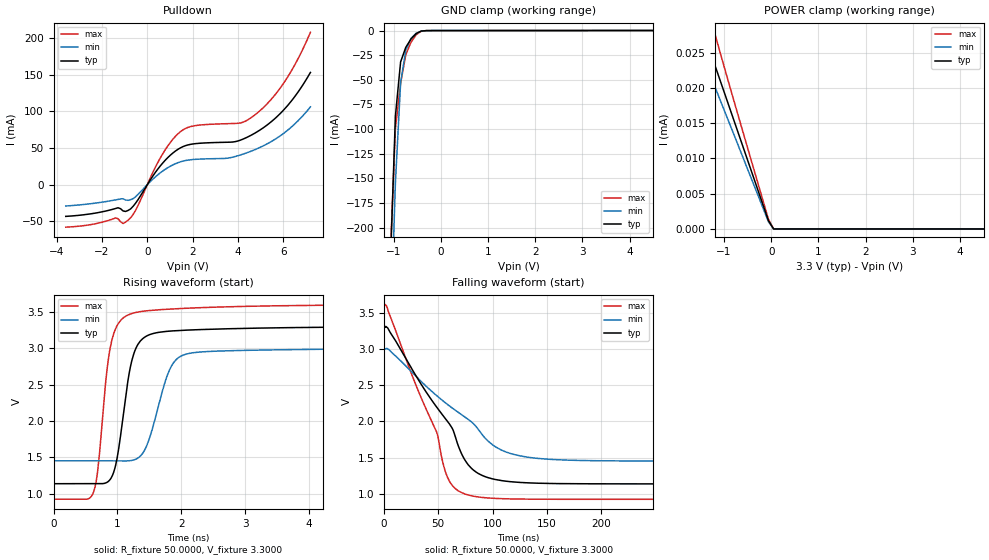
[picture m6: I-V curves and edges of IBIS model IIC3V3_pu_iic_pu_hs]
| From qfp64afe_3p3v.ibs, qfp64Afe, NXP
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[Model] IIC3V3_pu_iic_pu_hs
|   Model IIC3V3_pu_iic_pu_hs
| This model was characterised for following simulation conditions:
| External (pad) voltage:
|   - Typ: 3.3V,   - Min: 3.0V,   - Max: 3.6V
| Library cells for typ/min/max conditions are connected as defined below:
|  IO - External Pad
|  A - Core Input
|  EN - Output Buffer Enable
|  BOOST - vdde
|  ECS - vdd
|  EGP - gnd
|  ENZI - vdd
|  EPD - gnd
|  EPUN - gnd
|  SSEL - vdd
|  ZI - NC
|  ZIF - NC
|  gnd - gnd
|  gnde - gnde
|  vdd - vdd
|  vdde - vdde
| All other pins connected to ground
Model_type I/O_open_drain
Polarity   Non-Inverting
Enable   Active-Low
Vinl =   0.9900V
Vinh =   2.3100V
Vmeas =  1.6500V
Cref =   0.0F
Rref =   1.0000k
Vref =   3.3000V
C_comp   3.5867pF   3.4362pF   3.7352pF
|C_comp_pullup   0.9044pF   0.8908pF   0.9076pF
|C_comp_pulldown   2.3321pF   2.4859pF   2.1859pF
[Model Spec]
| variable   typ   min   max
Vinh   0.9900V   0.9000V   1.0800V
Vinl   2.3100V   2.1000V   2.5200V
Vmeas   1.6500V   1.5000V   1.8000V
Vref   3.3000V   3.0000V   3.6000V
Cref   0.0F   0.0F   0.0F
Rref   1.0000k   1.0000k   1.0000k
[Temperature Range]   25.0000   0.1250k   -40.0000
[Voltage Range]   3.3000V   3.0000V   3.6000V
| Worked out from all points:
|   slope of the pulldown table from 0 to 0.495 V, typ, clamps not added: 22 ohm
|   GND clamp passes 1 mA (typ) near -0.43 V on its own axis
|   rising waveform, R_fixture 50.0000, V_fixture 3.3000: 20-80 % time 227ps typ, 308ps min, 192ps max; typ from 1.14 V to 3.3 V
|   falling waveform, R_fixture 50.0000, V_fixture 3.3000: 20-80 % time 50.8ns typ, 68.7ns min, 38.5ns max; typ from 3.3 V to 1.14 V
[Pulldown]
|Voltage   I(typ)   I(min)   I(max)
-3.6V     -43.22mA   -29.09mA   -57.9mA
-1.29V    -31.46mA   -20.15mA   -46.47mA
-1.07V    -35.79mA   -19.19mA   -52.9mA
-850mV    -35.14mA   -21.36mA   -48.43mA
-520mV    -25.35mA   -16.52mA   -35.11mA
580mV     25.81mA    16.3mA     36.8mA
1.24V     45.79mA    28.53mA    65.82mA
1.9V      54.89mA    33.9mA     79.08mA
4.1V      60.55mA    40.38mA    84.05mA
4.76V     70.44mA    47.87mA    95.32mA
6.08V     103.9mA    71.39mA    141.2mA
7.2V      152.9mA    106mA      207.6mA
[GND_clamp]
|Voltage   I(typ)   I(min)   I(max)
-3.6V     -5.602A    -5.487A    -5.717A
-1.07V    -242.1mA   -316.8mA   -230.6mA
-960mV    -86.82mA   -154.8mA   -99.57mA
-850mV    -31.89mA   -53.14mA   -53.6mA
-740mV    -17.03mA   -19.92mA   -24.52mA
-630mV    -8.661mA   -7.977mA   -11.97mA
-520mV    -3.068mA   -2.784mA   -4.278mA
-410mV    -504.1uA   -552.6uA   -671.9uA
7.2V      0A         0A         0A
[POWER_clamp]
|Voltage   I(typ)   I(min)   I(max)
-3.6V     71.92uA    60.65uA    145.6uA
-1.71V    33.28uA    28.87uA    40.89uA
-1.6V     31.13uA    27.02uA    37.92uA
-1.49V    28.99uA    25.16uA    35.04uA
-1.38V    26.85uA    23.31uA    32.26uA
-1.27V    24.71uA    21.46uA    29.54uA
-1.16V    22.58uA    19.61uA    26.88uA
-720mV    14.02uA    12.19uA    16.54uA
-60mV     1.171uA    1.025uA    1.377uA
50mV      0A         0A         0A
7.2V      0A         0A         0A
[Ramp]
| variable   typ   min   max
dV/dt_r  1.2984/0.2267n   0.9292/0.3085n   1.6064/0.1919n
dV/dt_f  1.2984/50.8009n   0.9292/68.6899n   1.6064/38.4901n
R_load = 50.0000
[Rising Waveform]
R_fixture= 50.0000
V_fixture= 3.3000
V_fixture_min= 3.0000
V_fixture_max= 3.6000
|time   V(typ)   V(min)   V(max)
0s        1.136V     1.451V     922.6mV
623.4ps   1.136V     1.451V     1.014V
886ps     1.194V     1.451V     2.998V
993.8ps   1.479V     1.45V      3.308V
1.153ns   2.48V      1.45V      3.45V
1.388ns   3.124V     1.545V     3.506V
1.814ns   3.234V     2.698V     3.537V
2.038ns   3.246V     2.907V     3.547V
5.627ns   3.295V     2.993V     3.596V
1us       3.3V       3V         3.6V
[Falling Waveform]
R_fixture= 50.0000
V_fixture= 3.3000
V_fixture_min= 3.0000
V_fixture_max= 3.6000
|time   V(typ)   V(min)   V(max)
0s        3.3V       3V         3.6V
2.47ns    3.303V     3.01V      3.593V
48.48ns   2.199V     2.357V     1.853V
54.57ns   2.077V     2.281V     1.408V
59.76ns   1.976V     2.22V      1.187V
73.85ns   1.483V     2.068V     1.001V
83.34ns   1.316V     1.955V     963.2mV
112.4ns   1.173V     1.577V     929.9mV
163.8ns   1.14V      1.468V     923.1mV
1us       1.136V     1.451V     922.6mV
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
